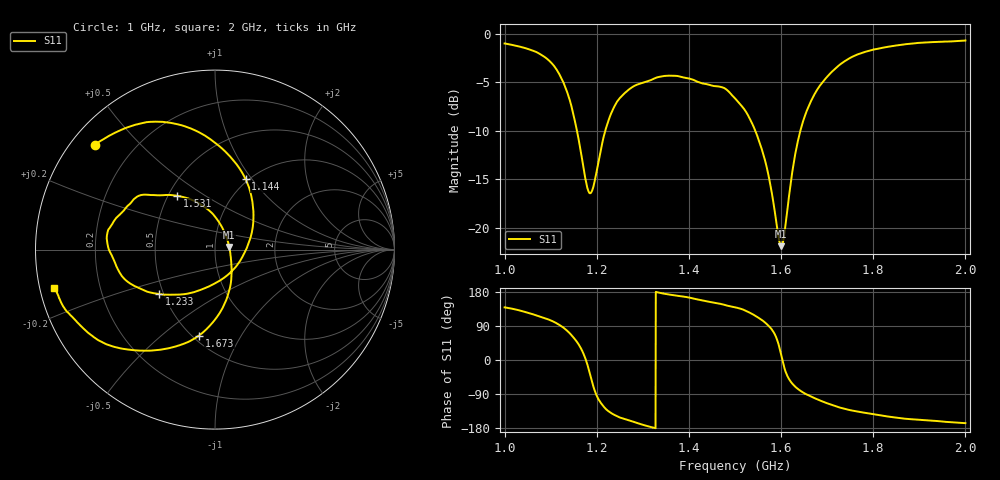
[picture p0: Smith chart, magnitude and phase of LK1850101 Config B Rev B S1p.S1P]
!Agilent Technologies,E5071C,MY46419360,A.11.08
!Date: Thu Sep 05 17:32:25 2024
!Data & Calibration Information:
!Freq	S11:SOLT1(ON)
!PortZ  Port1:50+j0
!Above PortZ is port z conversion or system Z0 setting when saving the data.
!When reading, reference impedance value at option line is always used.
# Hz S RI R 50
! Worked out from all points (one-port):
!   1601 points, 1 GHz to 2 GHz, reference 50 ohm
!   lowest |S11| = -21.9 dB at 1.601 GHz (marker M1), VSWR 1.17, Z = 58.5 + j1.8 ohm
!   |S11| at or under -10 dB: 1.157 GHz to 1.218 GHz (61.48 MHz wide, 5.18 % of centre); 1.544 GHz to 1.642 GHz (97.93 MHz wide, 6.15 % of centre)
!   S11 on the Smith chart (normalised r, x): 1 GHz: 0.07, +0.37; 1.144 GHz: 0.97, +0.93; 1.233 GHz: 0.47, -0.28; 1.531 GHz: 0.55, +0.38; 1.673 GHz: 0.54, -0.68; 2 GHz: 0.04, -0.12
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1e9  -0.6697 0.5851
1.034375e9  -0.5515 0.6538
1.07875e9  -0.3178 0.7123
1.104375e9  -0.1465 0.6792
1.125e9  0.0232 0.5772
1.144375e9  0.1704 0.3928
1.164375e9  0.2124 0.1406
1.1775e9  0.1678 -0.011
1.185625e9  0.1172 -0.0944
1.20875e9  -0.0991 -0.2307
1.233125e9  -0.3108 -0.2475
1.25e9  -0.4098 -0.2207
1.3e9  -0.5513 -0.0874
1.375e9  -0.5948 0.1099
1.46875e9  -0.4514 0.2816
1.5e9  -0.3504 0.3039
1.53125e9  -0.2124 0.3003
1.565625e9  -0.0323 0.2179
1.594375e9  0.0669 0.0604
1.600625e9  0.0789 0.0153
1.6075e9  0.0873 -0.0358
1.625e9  0.0894 -0.1772
1.645e9  0.0375 -0.3346
1.6725e9  -0.0891 -0.4788
1.706875e9  -0.286 -0.5551
1.75e9  -0.5055 -0.5541
1.875e9  -0.8058 -0.365
2e9  -0.8969 -0.2142
